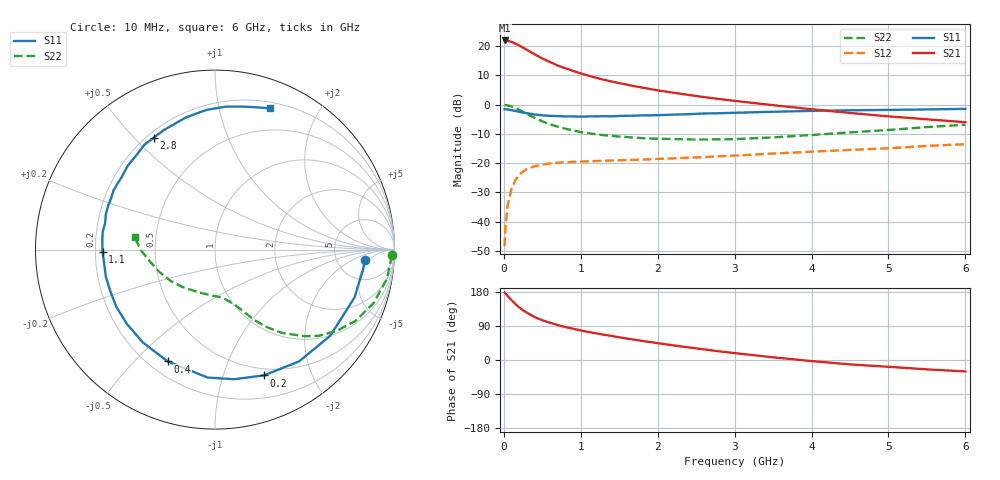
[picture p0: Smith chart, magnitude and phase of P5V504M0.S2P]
! SIEMENS Small Signal Semiconductors
! BFP183
! Si NPN RF Bipolar Junction Transistor in SOT143
! VCE = 0.5 V  IC = 4 mA
! Common Emitter S-Parameters:  March  1996
# GHz  S  MA  R  50
!  f  S11  S21  S12  S22
! GHz  MAG  ANG  MAG  ANG  MAG  ANG  MAG  ANG
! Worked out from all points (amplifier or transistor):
!   36 points, 10 MHz to 6 GHz, reference 50 ohm
!   highest |S21| = 21.9 dB at 10 MHz (marker M1)
!   |S21| within 3 dB of that: start of sweep to 285.1 MHz
!   unconditionally stable (mu >= 1): 1.504 GHz to end of sweep
!   at 250 MHz: K = 0.20, MSG = 21.2 dB, |S12| = -22.9 dB
!   at 1.4 GHz: K = 0.96, MSG = 13.5 dB, |S12| = -19.1 dB
!   at 6 GHz: K = 1.17, MAG = 1.3 dB, |S12| = -13.6 dB
!   S11 on the Smith chart (normalised r, x): 10 MHz: 10, -4; 200 MHz: 0.43, -1.37; 400 MHz: 0.27, -0.63; 1.1 GHz: 0.23, -0.01; 2.8 GHz: 0.23, +0.57; 6 GHz: 0.26, +1.43
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0.01  0.8359 -3.9  12.48 177.9  0.0038 84.0  0.9878 -1.9
0.02  0.8327 -7.5  12.41 175.9  0.0078 87.5  0.9803 -3.9
0.05  0.8218 -18.9  12.35 168.6  0.0192 80.2  0.9719 -9.6
0.1  0.8018 -36.8  11.76 157.7  0.0361 70.1  0.9315 -18.8
0.15  0.7794 -53.1  11.03 147.7  0.0511 62.0  0.8781 -26.9
0.2  0.7518 -68.8  10.29 138.6  0.0632 55.3  0.8142 -33.9
0.25  0.7298 -81.7  9.372 131.0  0.0719 49.1  0.7508 -39.8
0.3  0.714 -93.3  8.614 124.8  0.0794 44.3  0.6934 -44.1
0.4  0.6766 -112.9  7.242 113.4  0.0886 36.9  0.5944 -51.3
0.5  0.6551 -127.8  6.129 104.9  0.0945 31.5  0.5167 -56.4
0.6  0.6423 -139.7  5.341 98.2  0.0986 27.9  0.461 -60.0
0.7  0.6357 -149.7  4.658 92.3  0.1011 25.1  0.4191 -62.6
0.9  0.6268 -165.9  3.761 82.5  0.1052 21.9  0.3607 -66.9
1.1  0.6268 -178.9  3.119 73.8  0.1073 19.6  0.3229 -70.7
1.5  0.6389 162.3  2.324 59.8  0.1116 17.8  0.2841 -77.8
1.8  0.6543 149.7  1.95 50.3  0.1151 18.1  0.2671 -83.9
2.2  0.6742 136.1  1.598 38.7  0.1205 17.6  0.2577 -93.2
2.8  0.711 118.6  1.246 22.8  0.131 17.9  0.2543 -109.7
3.5  0.754 102.4  0.977 7.1  0.1455 16.9  0.2751 -130.0
4.5  0.7992 85.5  0.719 -11.6  0.1681 13.4  0.3347 -158.3
5.5  0.8262 73.6  0.56 -24.7  0.1968 9.4  0.4128 -179.4
6  0.8453 68.6  0.5 -30.2  0.2101 5.7  0.4527 171.2
